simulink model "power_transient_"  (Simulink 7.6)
settings: Solver=ode23tb  SolverMode=SingleTasking  StartTime=0.0  StopTime=0.2  RelTol=1e-4
InitFcn:
  | clc
StopFcn:
  | close all
  | load phasor.mat
  | subplot 211
  | plot(x(1,:),x(2,:))
  | title('Phaseur tension')
  | grid
  | 
  | subplot 212
  | plot (x(1,:),x(3,:))
  | axis([0 0.2 -200 800])
  | title('Phaseur courant')
  | grid
  | xlabel('temps')
libraries: powerlib x15

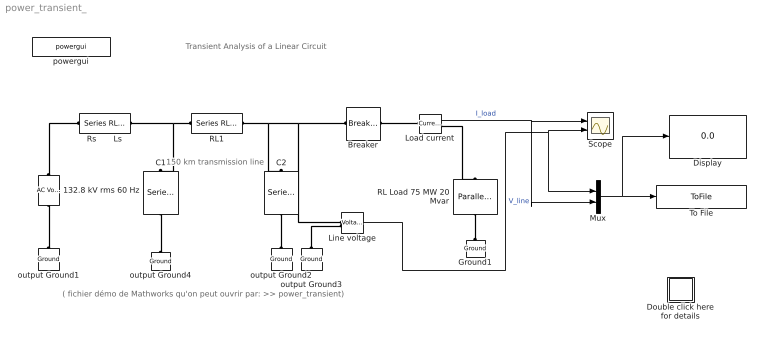
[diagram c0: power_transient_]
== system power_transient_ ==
  note: 150 km transmission line
  note: Transient Analysis of a Linear Circuit
  note: ( fichier démo de Mathworks qu'on peut ouvrir par: >> power_transient)
  132.8 kV rms 60 Hz : powerlib/Electrical Sources/AC Voltage Source  Description=source block  DialogController=POWERSYS.PowerSysDialog  SystemSampleTime=-1  Amplitude=230e3/sqrt(3)*sqrt(2)  Phase=90  Frequency=60  SampleTime=0  Measurements=None
  Breaker : powerlib/Elements/Breaker  DialogController=POWERSYS.PowerSysDialog  SystemSampleTime=-1  BreakerResistance=0.01  InitialState=1  SnubberResistance=inf  SnubberCapacitance=0  SwitchingTimes="[2/60  7/60 ]"  External=off  Measurements=None  MoreParameters=off  NoBreakLoop=off
  C1 : powerlib/Elements/Series RLC Branch  DialogController=POWERSYS.PowerSysDialog  PhysicalDomain=powersysdomain  SubClassName=unknown  LeftPortType=p1  RightPortType=p1  LConnTagsString=__new0  RConnTagsString=__new0  BranchType=C  Resistance=[]  Inductance=[]  SetiL0=off  InitialCurrent=0  Capacitance=0.967e-06  Setx0=off  InitialVoltage=0  Measurements=None
  C2 : powerlib/Elements/Series RLC Branch  DialogController=POWERSYS.PowerSysDialog  PhysicalDomain=powersysdomain  SubClassName=unknown  LeftPortType=p1  RightPortType=p1  LConnTagsString=__new0  RConnTagsString=__new0  BranchType=C  Resistance=[]  Inductance=[]  SetiL0=off  InitialCurrent=0  Capacitance=0.967e-06  Setx0=off  InitialVoltage=0  Measurements=None
  Display : Display
  Double click here for details : Subsystem
  Ground1 : powerlib/Elements/Ground  DialogController=POWERSYS.PowerSysDialog  PhysicalDomain=powersysdomain  SubClassName=unknown  LeftPortType=p1  RightPortType=p1  LConnTagsString=a
  Line voltage : powerlib/Measurements/Voltage Measurement  Tag=PoWeRsYsTeMmEaSuReMeNt  DialogController=POWERSYS.PowerSysDialog  SystemSampleTime=-1  PhasorSimulation=on  OutputType=Magnitude  PSBequivalent=0
  Load current : powerlib/Measurements/Current Measurement  Tag=PoWeRsYsTeMmEaSuReMeNt  DialogController=POWERSYS.PowerSysDialog  SystemSampleTime=-1  PhasorSimulation=on  OutputType=Magnitude  PSBequivalent=0
  Mux : Mux  Inputs=2
  RL Load 75 MW 20 Mvar : powerlib/Elements/Parallel RLC Load  DialogController=POWERSYS.PowerSysDialog  PhysicalDomain=powersysdomain  SubClassName=unknown  LeftPortType=p1  RightPortType=p1  LConnTagsString=a  RConnTagsString=__new0  NominalVoltage=132.8e3  NominalFrequency=60  ActivePower=75e6  InductivePower=20e6  CapacitivePower=0  Setx0=off  InitialVoltage=0  SetiL0=off  InitialCurrent=0  Measurements=None
  RL1 : powerlib/Elements/Series RLC Branch  DialogController=POWERSYS.PowerSysDialog  PhysicalDomain=powersysdomain  SubClassName=unknown  LeftPortType=p1  RightPortType=p1  LConnTagsString=__new0  RConnTagsString=__new0  BranchType=RL  Resistance=5.2  Inductance=138e-3  SetiL0=off  InitialCurrent=0  Capacitance=[]  Setx0=off  InitialVoltage=0  Measurements=None
  Rs       Ls : powerlib/Elements/Series RLC Branch  DialogController=POWERSYS.PowerSysDialog  PhysicalDomain=powersysdomain  SubClassName=unknown  LeftPortType=p1  RightPortType=p1  LConnTagsString=__new0  RConnTagsString=__new0  BranchType=RL  Resistance=2.645  Inductance=70.2e-03  SetiL0=off  InitialCurrent=0  Capacitance=[]  Setx0=off  InitialVoltage=0  Measurements=None
  Scope : Scope  NumInputPorts=2
  To File : ToFile  Filename=phasor.mat  MatrixName=x
  output Ground{1..4} (4 alike) : powerlib/Elements/Ground  DialogController=POWERSYS.PowerSysDialog  PhysicalDomain=powersysdomain  SubClassName=unknown  LeftPortType=p1  RightPortType=p1  LConnTagsString=a
  powergui : powerlib/powergui  Priority=2  SystemSampleTime=-1  SimulationMode=Phasor  SampleTime=0  frequency=60  SPID=off  DisableSnubberDevices=off  DisableRonSwitches=off  DisableVfSwitches=off  SwTol=0  Interpol=off  frequencyindice=60  echomessages=off  HookPort=off  DisplayEquations=off  FunctionMessages=off  EnableUseOfTLC=off  x0status=blocks  RestoreLinks=warning  ResistiveCurrentMeasurement=off  Frange=logspace(0,3,50)  Ylog=off  Xlog=off  ShowGrid=off  save=off  variable=ZData  ZoomFFT=on  StartTime=0.0  cycles=1  DisplayStyle=off  fundamental=60  FreqAxis=off  MaxFrequency=1000  frequencyindicesteady=1  RmsSteady=1  display=off  Ts=0  methode=off
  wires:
  Line voltage/1 -> Scope/2, Mux/1  "V_line"
  Load current/1 -> Scope/1, Mux/2  "I_load"
  Mux/1 -> To File/1, Display/1
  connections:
  RL Load 75 MW 20 Mvar/RConn1 -- Ground1/LConn1
  output Ground3/LConn1 -- Line voltage/LConn2
  RL1/RConn1 -- Line voltage/LConn1 -- Breaker/LConn1 -- C2/LConn1
  132.8 kV rms 60 Hz/RConn1 -- Rs       Ls/LConn1
  output Ground1/LConn1 -- 132.8 kV rms 60 Hz/LConn1
  Breaker/RConn1 -- Load current/LConn1
  Load current/RConn1 -- RL Load 75 MW 20 Mvar/LConn1
  RL1/LConn1 -- Rs       Ls/RConn1 -- C1/LConn1
  C1/RConn1 -- output Ground4/LConn1
  C2/RConn1 -- output Ground2/LConn1

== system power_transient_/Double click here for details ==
